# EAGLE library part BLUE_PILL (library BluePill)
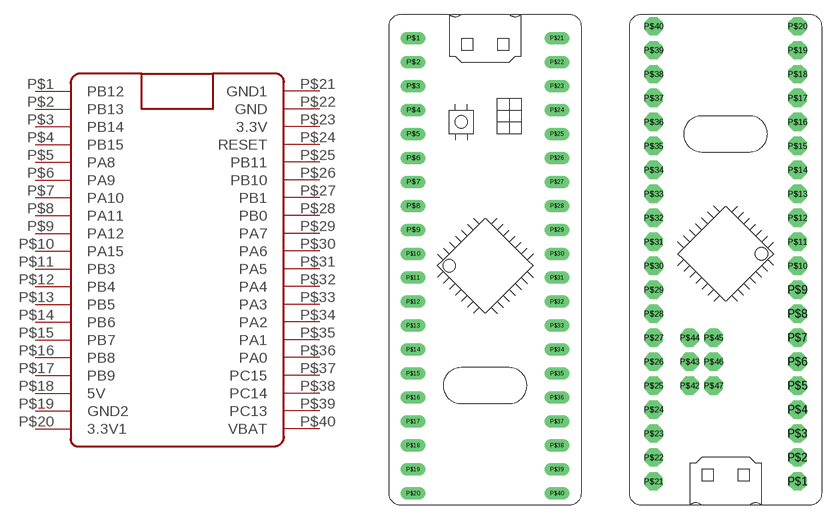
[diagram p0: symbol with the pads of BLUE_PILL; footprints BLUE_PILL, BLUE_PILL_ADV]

Designator prefix -

## BLUE_PILL  [BLUE_PILL]
P$1  PB12
P$2  PB13
P$3  PB14
P$4  PB15
P$5  PA8
P$6  PA9
P$7  PA10
P$8  PA11
P$9  PA12
P$10  PA15
P$11  PB3
P$12  PB4
P$13  PB5
P$14  PB6
P$15  PB7
P$16  PB8
P$17  PB9
P$18  5V
P$19  GND2
P$20  3.3V1
P$21  GND1  pwr
P$22  GND
P$23  3.3V
P$24  RESET
P$25  PB11
P$26  PB10
P$27  PB1
P$28  PB0
P$29  PA7
P$30  PA6
P$31  PA5
P$32  PA4
P$33  PA3
P$34  PA2
P$35  PA1
P$36  PA0
P$37  PC15
P$38  PC14
P$39  PC13
P$40  VBAT

## BLUE_PILLADVANCED  [BLUE_PILL_ADV]
Pads as for BLUE_PILL

## Footprint BLUE_PILL (pad centres in mm)
drill 0.8 long: P$1 -7.62,15.24; P$2 -7.62,12.7; P$3 -7.62,10.16; P$4 -7.62,7.62; P$5 -7.62,5.08; P$6 -7.62,2.54; P$7 -7.62,0; P$8 -7.62,-2.54; P$9 -7.62,-5.08; P$10 -7.62,-7.62; P$11 -7.62,-10.16; P$12 -7.62,-12.7; P$13 -7.62,-15.24; P$14 -7.62,-17.78; P$15 -7.62,-20.32; P$16 -7.62,-22.86; P$17 -7.62,-25.4; P$18 -7.62,-27.94; P$19 -7.62,-30.48; P$20 -7.62,-33.02; P$21 7.62,15.24; P$22 7.62,12.7; P$23 7.62,10.16; P$24 7.62,7.62; P$25 7.62,5.08; P$26 7.62,2.54; P$27 7.62,0; P$28 7.62,-2.54; P$29 7.62,-5.08; P$30 7.62,-7.62; P$31 7.62,-10.16; P$32 7.62,-12.7; P$33 7.62,-15.24; P$34 7.62,-17.78; P$35 7.62,-20.32; P$36 7.62,-22.86; P$37 7.62,-25.4; P$38 7.62,-27.94; P$39 7.62,-30.48; P$40 7.62,-33.02

## Footprint BLUE_PILL_ADV (pad centres in mm)
drill 0.8 pad 1.93 octagon: P$1 10.16,-30.48; P$2 10.16,-27.94; P$3 10.16,-25.4; P$4 10.16,-22.86; P$5 10.16,-20.32; P$6 10.16,-17.78; P$7 10.16,-15.24; P$8 10.16,-12.7; P$9 10.16,-10.16; P$10 10.16,-7.62; P$11 10.16,-5.08; P$12 10.16,-2.54; P$13 10.16,0; P$14 10.16,2.54; P$15 10.16,5.08; P$16 10.16,7.62; P$17 10.16,10.16; P$18 10.16,12.7; P$19 10.16,15.24; P$20 10.16,17.78; P$21 -5.08,-30.48; P$22 -5.08,-27.94; P$23 -5.08,-25.4; P$24 -5.08,-22.86; P$25 -5.08,-20.32; P$26 -5.08,-17.78; P$27 -5.08,-15.24; P$28 -5.08,-12.7; P$29 -5.08,-10.16; P$30 -5.08,-7.62; P$31 -5.08,-5.08; P$32 -5.08,-2.54; P$33 -5.08,0; P$34 -5.08,2.54; P$35 -5.08,5.08; P$36 -5.08,7.62; P$37 -5.08,10.16; P$38 -5.08,12.7; P$39 -5.08,15.24; P$40 -5.08,17.78
drill 1.1 pad 1.93 octagon: P$42 -1.27,-20.32; P$43 -1.27,-17.78; P$44 -1.27,-15.24; P$45 1.27,-15.24; P$46 1.27,-17.78; P$47 1.27,-20.32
